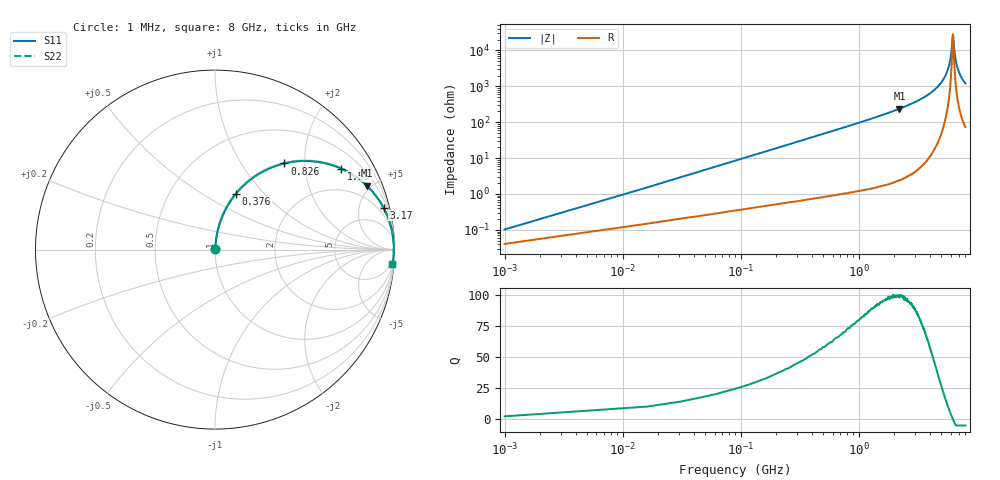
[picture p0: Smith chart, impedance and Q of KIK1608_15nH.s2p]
!version-2
!date-01.2022
!Series
# MHz S RI R 50
!Freq ReS11 ImS11 ReS21 ImS21 ReS12 ImS12 ReS22 ImS22
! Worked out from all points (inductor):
!   535 points, 1 MHz to 8 GHz, reference 50 ohm
!   read as one part in series: L = 15 nH near 31 MHz
!   highest Q = 99.3 at 2.21 GHz (marker M1), where L = 17.1 nH
!   self-resonance near 6.27 GHz
!   S11 on the Smith chart (normalised r, x): 1 MHz: 1.00, +0.00; 376 MHz: 1.01, +0.71; 826 MHz: 1.02, +1.58; 1.55 GHz: 1.03, +3.10; 3.17 GHz: 1.10, +8.01; 8 GHz: 2, -24
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1  0.000413 0.000942  0.9996 -0.000942  0.9996 -0.000942  0.000413 0.000942
46  0.00435 0.0431  0.9957 -0.0431  0.9957 -0.0431  0.00435 0.0431
91  0.0107 0.0846  0.9893 -0.0846  0.9893 -0.0846  0.0107 0.0846
196  0.0376 0.177  0.9624 -0.177  0.9624 -0.177  0.0376 0.177
376  0.1171 0.3118  0.8829 -0.3118  0.8829 -0.3118  0.1171 0.3118
826  0.3871 0.4803  0.6129 -0.4803  0.6129 -0.4803  0.3871 0.4803
1340  0.6336 0.4763  0.3664 -0.4763  0.3664 -0.4763  0.6336 0.4763
1550  0.7045 0.451  0.2955 -0.451  0.2955 -0.451  0.7045 0.451
2210  0.8466 0.3553  0.1534 -0.3553  0.1534 -0.3553  0.8466 0.3553
2670  0.9018 0.2923  0.0982 -0.2923  0.0982 -0.2923  0.9018 0.2923
3170  0.9388 0.2338  0.0612 -0.2338  0.0612 -0.2338  0.9388 0.2338
4010  0.9734 0.1523  0.0266 -0.1523  0.0266 -0.1523  0.9734 0.1523
5340  0.994 0.0543  0.00599 -0.0543  0.00599 -0.0543  0.994 0.0543
5690  0.9957 0.0332  0.0043 -0.0332  0.0043 -0.0332  0.9957 0.0332
5930  0.9963 0.0193  0.00371 -0.0193  0.00371 -0.0193  0.9963 0.0193
6080  0.9965 0.0109  0.00355 -0.0109  0.00355 -0.0109  0.9965 0.0109
6270  0.9964 0.000251  0.00356 -0.000251  0.00356 -0.000251  0.9964 0.000251
6320  0.9964 -0.00215  0.00359 0.00215  0.00359 0.00215  0.9964 -0.00215
6480  0.9962 -0.0108  0.00382 0.0108  0.00382 0.0108  0.9962 -0.0108
6680  0.9957 -0.0208  0.00428 0.0208  0.00428 0.0208  0.9957 -0.0208
7170  0.9937 -0.0447  0.00626 0.0447  0.00626 0.0447  0.9937 -0.0447
8000  0.9883 -0.0815  0.0117 0.0815  0.0117 0.0815  0.9883 -0.0815
